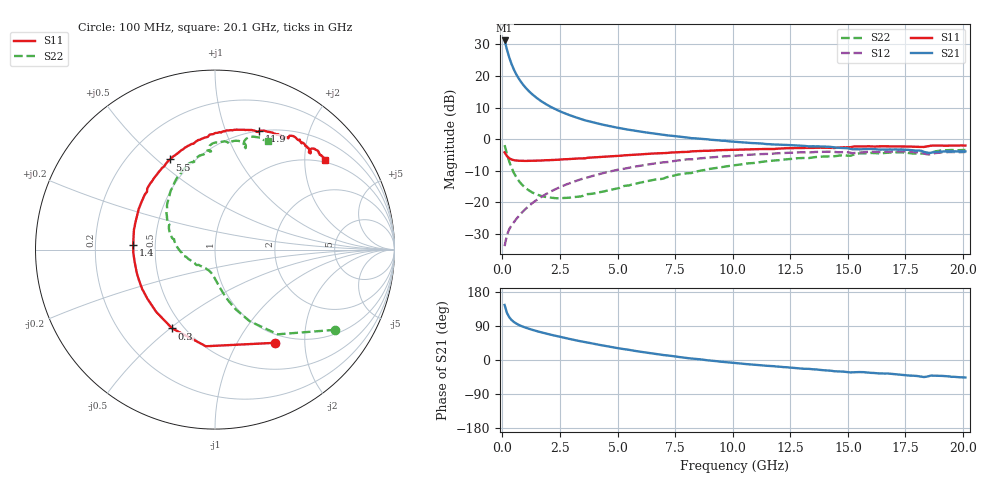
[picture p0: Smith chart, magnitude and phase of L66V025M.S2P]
!  Infineon Technologies AG
! BFR380L3 , PF131585-7, No.6, Th 09.10.01, soldered on pcb-board, measured with PP GSG850
!  Vce=6.0 V,  Ic=25.0 mA
! Common Emitter S-Parameters:  15. November 2001
#  GHz  S  MA  R  50
! f  S11  S21  S12  S22
! GHz  Mag  Ang  Mag  Ang  Mag  Ang  Mag  Ang
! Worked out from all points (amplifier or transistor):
!   201 points, 100 MHz to 20.1 GHz, reference 50 ohm
!   highest |S21| = 31.2 dB at 100 MHz (marker M1)
!   |S21| within 3 dB of that: start of sweep to 206.7 MHz
!   unconditionally stable (mu >= 1): 1.367 GHz to 4.379 GHz
!   at 3.4 GHz: K = 1.02, MAG = 8.7 dB, |S12| = -12.7 dB
!   at 10.1 GHz: K = 0.95, MSG = 2.2 dB, |S12| = -5.2 dB
!   at 20.1 GHz: K = 0.98, MSG = 0.1 dB, |S12| = -4.1 dB
!   S11 on the Smith chart (normalised r, x): 100 MHz: 0.87, -1.46; 300 MHz: 0.43, -0.51; 1.4 GHz: 0.37, +0.02; 5.5 GHz: 0.38, +0.55; 11.9 GHz: 0.50, +1.32; 20.1 GHz: 0.94, +2.51
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0.1  0.6179 -57.2  36.3 145.2  0.02037 64.3  0.8061 -33.7
0.2  0.5409 -95.4  26.2 124.5  0.03046 57.2  0.5875 -53.5
0.3  0.4997 -118.5  19.6 113.1  0.03781 55.2  0.4435 -64.2
0.4  0.4773 -133.3  15.43 105.6  0.0433 55.7  0.3533 -70.8
0.5  0.4655 -144.1  12.64 100.4  0.04864 57.1  0.2942 -75.3
0.6  0.461 -152.0  10.68 96.5  0.05439 58.6  0.2534 -78.7
0.7  0.4564 -158.2  9.248 93.2  0.06005 59.9  0.2231 -81.6
0.8  0.4548 -163.3  8.15 90.3  0.06626 61.4  0.2008 -84.0
0.9  0.4528 -167.6  7.277 87.9  0.07223 62.3  0.1836 -86.1
1.1  0.4538 -174.7  6.008 83.5  0.08476 63.5  0.16 -90.5
1.4  0.4563 176.8  4.766 77.9  0.1037 64.3  0.1381 -96.2
1.8  0.4618 168.0  3.748 71.3  0.1295 64.1  0.1234 -104.2
2.2  0.4689 160.5  3.106 65.4  0.1553 62.9  0.118 -112.7
2.8  0.4824 150.6  2.489 57.1  0.1935 60.4  0.1181 -125.4
3.5  0.4971 140.1  2.033 48.2  0.238 56.7  0.1271 -137.8
5.5  0.5615 116.6  1.408 26.8  0.3532 44.3  0.1858 -174.8
6.8  0.5988 103.7  1.195 14.6  0.4227 35.4  0.234 166.7
10.1  0.68 79.1  0.9092 -7.8  0.5503 13.9  0.3885 131.6
11.9  0.7058 69.5  0.8243 -17.1  0.5971 3.0  0.4618 115.0
13.5  0.728 61.4  0.7731 -24.6  0.6232 -7.1  0.5148 102.7
16.8  0.7688 48.6  0.6881 -36.0  0.633 -23.5  0.6126 80.6
20.1  0.7916 39.1  0.6411 -46.2  0.6271 -37.4  0.6749 63.9
